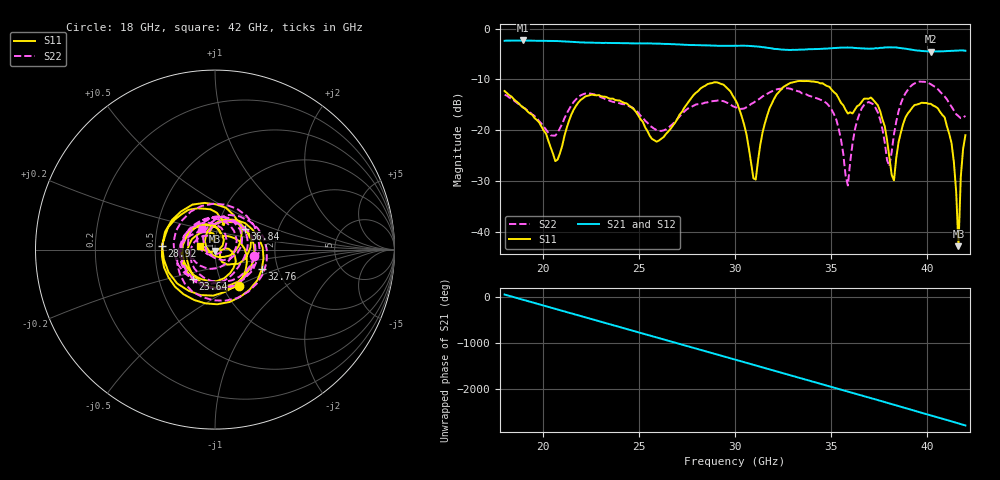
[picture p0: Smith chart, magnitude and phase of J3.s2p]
!Agilent Technologies,N5230A,US43500212,A.07.50.67
!Agilent N5230A: A.07.50.67
!Date: Monday, September 22, 2025 06:01:52
!Correction: S11(Full 2 Port(1,2))
!S21(Full 2 Port(1,2))
!S12(Full 2 Port(1,2))
!S22(Full 2 Port(1,2))
!S2P File: Measurements: S11, S21, S12, S22:
# Hz S  dB  R 50
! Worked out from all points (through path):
!   201 points, 18 GHz to 42 GHz, reference 50 ohm
!   highest |S21| = -2.34 dB at 18.96 GHz (marker M1); lowest = -4.5 dB at 40.2 GHz (marker M2)
!   lowest |S11| = -42.9 dB at 41.64 GHz (marker M3), VSWR 1.01, Z = 50 - j0.716 ohm
!   |S11| at or under -10 dB: start of sweep to end of sweep
!   |S22| runs from -30.9 to -10.5 dB; largest |S21 - S12| = 0.0055
!   S11 on the Smith chart (normalised r, x): 18 GHz: 1.19, -0.51; 23.64 GHz: 0.74, -0.25; 28.92 GHz: 0.54, +0.03; 32.76 GHz: 1.65, -0.39; 36.84 GHz: 1.36, +0.33; 42 GHz: 0.84, +0.04
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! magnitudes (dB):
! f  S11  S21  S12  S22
! 18 GHz  -12.3  -2.4  -2.4  -13.0
! 18.96 GHz  -15.5  -2.3  -2.4  -15.5
! 20.64 GHz  -26.1  -2.4  -2.4  -21.1
! 22.08 GHz  -13.7  -2.7  -2.7  -13.0
! 23.64 GHz  -13.8  -2.8  -2.8  -14.4
! 26.04 GHz  -22.1  -3.0  -3.0  -20.1
! 28.92 GHz  -10.6  -3.4  -3.4  -14.3
! 30 GHz  -13.9  -3.4  -3.4  -15.5
! 31.08 GHz  -29.8  -3.5  -3.5  -14.3
! 32.76 GHz  -11.0  -4.2  -4.2  -11.8
! 34.08 GHz  -10.4  -4.1  -4.1  -13.5
! 35.28 GHz  -12.9  -3.8  -3.8  -18.0
! 35.88 GHz  -16.7  -3.7  -3.7  -30.9
! 36.84 GHz  -13.8  -4.0  -3.9  -14.7
! 38.04 GHz  -25.4  -3.7  -3.7  -27.2
! 38.28 GHz  -29.9  -3.7  -3.7  -20.8
! 38.76 GHz  -18.8  -3.9  -3.9  -13.6
! 40.2 GHz  -14.8  -4.5  -4.5  -11.0
! 41.28 GHz  -22.6  -4.4  -4.4  -15.4
! 41.64 GHz  -42.9  -4.3  -4.3  -17.3
! 41.76 GHz  -29.2  -4.3  -4.4  -17.7
! 42 GHz  -21.0  -4.4  -4.3  -17.2
